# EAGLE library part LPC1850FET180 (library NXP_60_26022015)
32-bit ARM Cortex-M3 MCU; up to 200 kB SRAM; Ethernet, two High-speed USB, LCD, and external memory controller The LPC1850/30/20/10 are ARM Cortex-M3 based microcontrollers for embedded applications. The ARM Cortex-M3 is a next generation core that offers system enhancements such as low power consumption, enhanced debug features, and a high level of support block integration. The LPC1850/30/20/10 operate at CPU frequencies of up to 180 MHz. The ARM Cortex-M3 CPU incorporates a 3-stage pipeline and uses a Harvard architecture with separate local instruction and data buses as well as a third bus for peripherals. The ARM Cortex-M3 CPU also includes an internal prefetch unit that supports speculative branching. The LPC1850/30/20/10 include up to 200 kB of on-chip SRAM, a quad SPI Flash Interface (SPIFI), a State Configurable Timer (SCT) subsystem, two High-speed USB controllers, Ethernet, LCD, an external memory controller, and multiple digital and analog peripherals. AAL Eindhoven MK
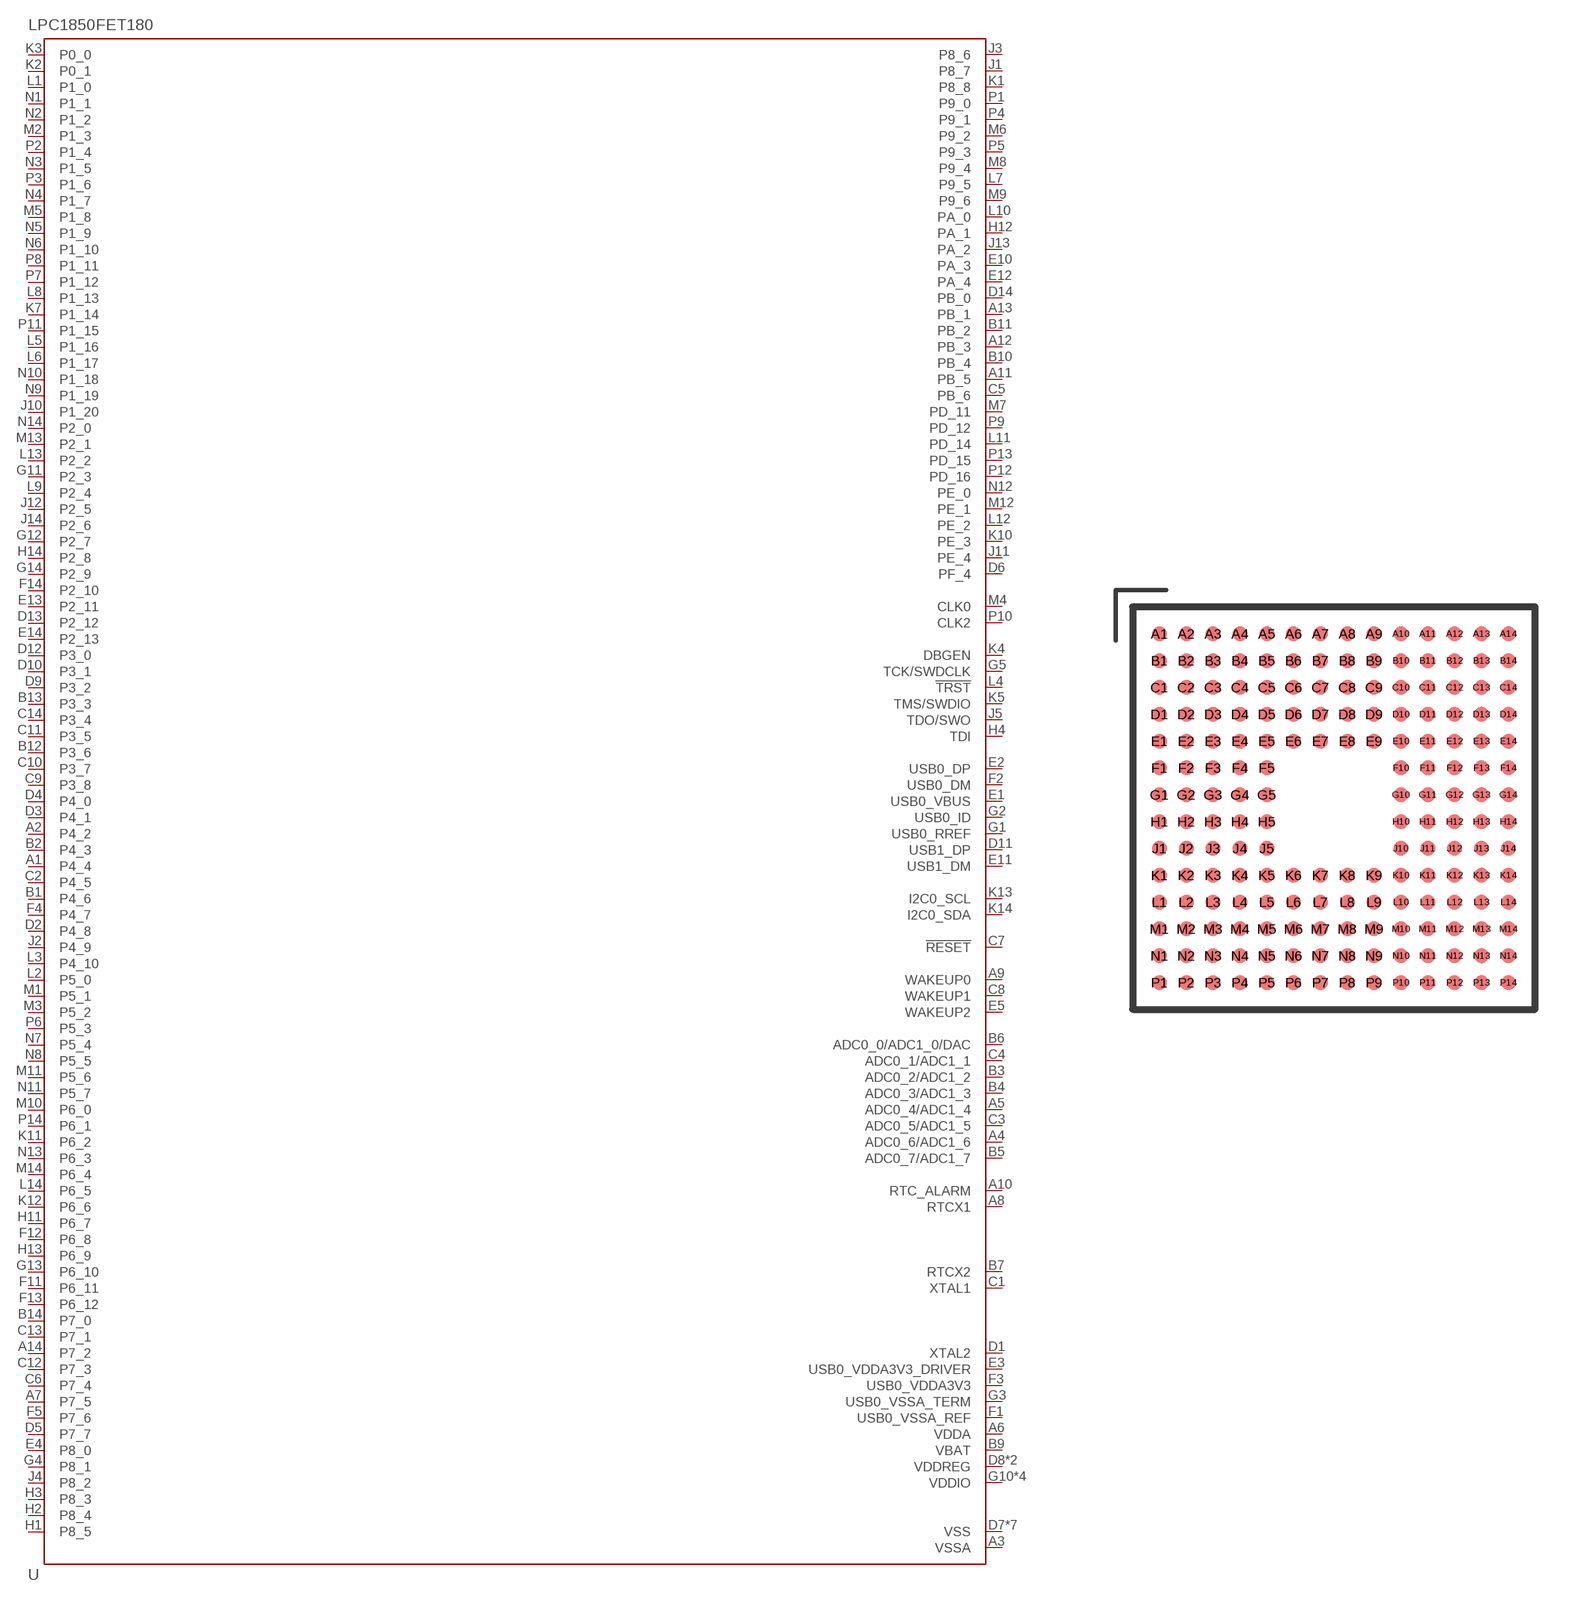
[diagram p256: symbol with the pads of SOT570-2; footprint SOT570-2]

Designator prefix U

## LPC1850FET180 (ADC: 8; ETHERNET: yes; GPIO: 118; LCD: yes; PWM: yes; QEI: yes; SRAM: 2000kB; USB0: Host/OTG; USB1: Host/ULPI)  [SOT570-2]
A1  P4_4
A2  P4_2
A3  VSSA
A4  ADC0_6/ADC1_6
A5  ADC0_4/ADC1_4
A6  VDDA
A7  P7_5
A8  RTCX1
A9  WAKEUP0
A10  RTC_ALARM
A11  PB_5
A12  PB_3
A13  PB_1
A14  P7_2
B1  P4_6
B2  P4_3
B3  ADC0_2/ADC1_2
B4  ADC0_3/ADC1_3
B5  ADC0_7/ADC1_7
B6  ADC0_0/ADC1_0/DAC
B7  RTCX2
B9  VBAT
B10  PB_4
B11  PB_2
B12  P3_6
B13  P3_3
B14  P7_0
C1  XTAL1
C2  P4_5
C3  ADC0_5/ADC1_5
C4  ADC0_1/ADC1_1
C5  PB_6
C6  P7_4
C7  !RESET
C8  WAKEUP1
C9  P3_8
C10  P3_7
C11  P3_5
C12  P7_3
C13  P7_1
C14  P3_4
D1  XTAL2
D2  P4_8
D3  P4_1
D4  P4_0
D5  P7_7
D6  PF_4
D7  VSS
D8  VDDREG
D9  P3_2
D10  P3_1
D11  USB1_DP
D12  P3_0
D13  P2_12
D14  PB_0
E1  USB0_VBUS
E2  USB0_DP
E3  USB0_VDDA3V3_DRIVER
E4  P8_0
E5  WAKEUP2
E6  VSS
E7  VSS
E8  VDDREG
E9  VSS
E10  PA_3
E11  USB1_DM
E12  PA_4
E13  P2_11
E14  P2_13
F1  USB0_VSSA_REF
F2  USB0_DM
F3  USB0_VDDA3V3
F4  P4_7
F5  P7_6
F10  VSS
F11  P6_11
F12  P6_8
F13  P6_12
F14  P2_10
G1  USB0_RREF
G2  USB0_ID
G3  USB0_VSSA_TERM
G4  P8_1
G5  TCK/SWDCLK
G10  VDDIO
G11  P2_3
G12  P2_7
G13  P6_10
G14  P2_9
H1  P8_5
H2  P8_4
H3  P8_3
H4  TDI
H5  VDDIO
H10  VDDIO
H11  P6_7
H12  PA_1
H13  P6_9
H14  P2_8
J1  P8_7
J2  P4_9
J3  P8_6
J4  P8_2
J5  TDO/SWO
J10  P1_20
J11  PE_4
J12  P2_5
J13  PA_2
J14  P2_6
K1  P8_8
K2  P0_1
K3  P0_0
K4  DBGEN
K5  TMS/SWDIO
K6  VSS
K7  P1_14
K8  VDDIO
K9  VSS
K10  PE_3
K11  P6_2
K12  P6_6
K13  I2C0_SCL
K14  I2C0_SDA
L1  P1_0
L2  P5_0
L3  P4_10
L4  !TRST
L5  P1_16
L6  P1_17
L7  P9_5
L8  P1_13
L9  P2_4
L10  PA_0
L11  PD_14
L12  PE_2
L13  P2_2
L14  P6_5
M1  P5_1
M2  P1_3
M3  P5_2
M4  CLK0
M5  P1_8
M6  P9_2
M7  PD_11
M8  P9_4
M9  P9_6
M10  P6_0
M11  P5_6
M12  PE_1
M13  P2_1
M14  P6_4
N1  P1_1
N2  P1_2
N3  P1_5
N4  P1_7
N5  P1_9
N6  P1_10
N7  P5_4
N8  P5_5
N9  P1_19
N10  P1_18
N11  P5_7
N12  PE_0
N13  P6_3
N14  P2_0
P1  P9_0
P2  P1_4
P3  P1_6
P4  P9_1
P5  P9_3
P6  P5_3
P7  P1_12
P8  P1_11
P9  PD_12
P10  CLK2
P11  P1_15
P12  PD_16
P13  PD_15
P14  P6_1

## Footprint SOT570-2 (pad centres in mm)
SOT570-2 TFBGA180: thin fine-pitch ball grid array package; 180 balls; body 12 x 12 x 0.8 mm JEDEC: -- IEC: -- JEITA: -- Shamelessly copied from nxp_packages.lbr
smd 0.45 x 0.45: A1 -5.2,5.2; A2 -4.4,5.2; A3 -3.6,5.2; A4 -2.8,5.2; A5 -2,5.2; A6 -1.2,5.2; A7 -0.4,5.2; A8 0.4,5.2; A9 1.2,5.2; A10 2,5.2; A11 2.8,5.2; A12 3.6,5.2; A13 4.4,5.2; A14 5.2,5.2; B1 -5.2,4.4; B2 -4.4,4.4; B3 -3.6,4.4; B4 -2.8,4.4; B5 -2,4.4; B6 -1.2,4.4; B7 -0.4,4.4; B8 0.4,4.4; B9 1.2,4.4; B10 2,4.4; B11 2.8,4.4; B12 3.6,4.4; B13 4.4,4.4; B14 5.2,4.4; C1 -5.2,3.6; C2 -4.4,3.6; C3 -3.6,3.6; C4 -2.8,3.6; C5 -2,3.6; C6 -1.2,3.6; C7 -0.4,3.6; C8 0.4,3.6; C9 1.2,3.6; C10 2,3.6; C11 2.8,3.6; C12 3.6,3.6; C13 4.4,3.6; C14 5.2,3.6; D1 -5.2,2.8; D2 -4.4,2.8; D3 -3.6,2.8; D4 -2.8,2.8; D5 -2,2.8; D6 -1.2,2.8; D7 -0.4,2.8; D8 0.4,2.8; D9 1.2,2.8; D10 2,2.8; D11 2.8,2.8; D12 3.6,2.8; D13 4.4,2.8; D14 5.2,2.8; E1 -5.2,2; E2 -4.4,2; E3 -3.6,2; E4 -2.8,2; E5 -2,2; E6 -1.2,2; E7 -0.4,2; E8 0.4,2; E9 1.2,2; E10 2,2; E11 2.8,2; E12 3.6,2; E13 4.4,2; E14 5.2,2; F1 -5.2,1.2; F2 -4.4,1.2; F3 -3.6,1.2; F4 -2.8,1.2; F5 -2,1.2; F10 2,1.2; F11 2.8,1.2; F12 3.6,1.2; F13 4.4,1.2; F14 5.2,1.2; G1 -5.2,0.4; G2 -4.4,0.4; G3 -3.6,0.4; G4 -2.8,0.4; G5 -2,0.4; G10 2,0.4; G11 2.8,0.4; G12 3.6,0.4; G13 4.4,0.4; G14 5.2,0.4; H1 -5.2,-0.4; H2 -4.4,-0.4; H3 -3.6,-0.4; H4 -2.8,-0.4; H5 -2,-0.4; H10 2,-0.4; H11 2.8,-0.4; H12 3.6,-0.4; H13 4.4,-0.4; H14 5.2,-0.4; J1 -5.2,-1.2; J2 -4.4,-1.2; J3 -3.6,-1.2; J4 -2.8,-1.2; J5 -2,-1.2; J10 2,-1.2; J11 2.8,-1.2; J12 3.6,-1.2; J13 4.4,-1.2; J14 5.2,-1.2; K1 -5.2,-2; K2 -4.4,-2; K3 -3.6,-2; K4 -2.8,-2; K5 -2,-2; K6 -1.2,-2; K7 -0.4,-2; K8 0.4,-2; K9 1.2,-2; K10 2,-2; K11 2.8,-2; K12 3.6,-2; K13 4.4,-2; K14 5.2,-2; L1 -5.2,-2.8; L2 -4.4,-2.8; L3 -3.6,-2.8; L4 -2.8,-2.8; L5 -2,-2.8; L6 -1.2,-2.8; L7 -0.4,-2.8; L8 0.4,-2.8; L9 1.2,-2.8; L10 2,-2.8; L11 2.8,-2.8; L12 3.6,-2.8; L13 4.4,-2.8; L14 5.2,-2.8; M1 -5.2,-3.6; M2 -4.4,-3.6; M3 -3.6,-3.6; M4 -2.8,-3.6; M5 -2,-3.6; M6 -1.2,-3.6; M7 -0.4,-3.6; M8 0.4,-3.6; M9 1.2,-3.6; M10 2,-3.6; M11 2.8,-3.6; M12 3.6,-3.6; M13 4.4,-3.6; M14 5.2,-3.6; N1 -5.2,-4.4; N2 -4.4,-4.4; N3 -3.6,-4.4; N4 -2.8,-4.4; N5 -2,-4.4; N6 -1.2,-4.4; N7 -0.4,-4.4; N8 0.4,-4.4; N9 1.2,-4.4; N10 2,-4.4; N11 2.8,-4.4; N12 3.6,-4.4; N13 4.4,-4.4; N14 5.2,-4.4; P1 -5.2,-5.2; P2 -4.4,-5.2; P3 -3.6,-5.2; P4 -2.8,-5.2; P5 -2,-5.2; P6 -1.2,-5.2; P7 -0.4,-5.2; P8 0.4,-5.2; P9 1.2,-5.2; P10 2,-5.2; P11 2.8,-5.2; P12 3.6,-5.2; P13 4.4,-5.2; P14 5.2,-5.2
